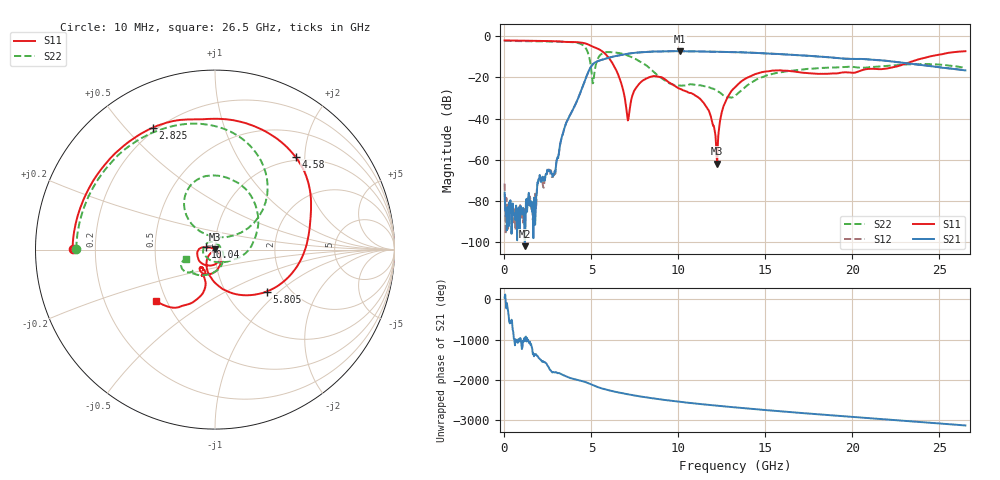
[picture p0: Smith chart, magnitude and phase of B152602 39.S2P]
!  2-Port S-parameters saved by WinCal
! VAR MeasName=S-Parameters (CALIBRATED_DATA) read from VNA (N5242A)
! VAR MeasDate=2016-1-5 16:31:50
! VAR NAME=B152602 39
! VAR FILENAME=B152602 39.S2P
! VAR DATE=2016-1-5 16:31:50
! VAR PHYS_PORTS=1,2
# Hz S DB R 50
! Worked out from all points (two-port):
!   801 points, 10 MHz to 26.5 GHz, reference 50 ohm
!   highest |S21| = -7.22 dB at 10.11 GHz (marker M1); lowest = -102.1 dB at 1.169 GHz (marker M2)
!   |S21| within 3 dB of the highest: 6.073 GHz to 18.7 GHz (12.62 GHz wide, 102 % of centre)
!   lowest |S11| = -61.9 dB at 12.23 GHz (marker M3), VSWR 1.00, Z = 50 + j0.0703 ohm
!   |S11| at or under -10 dB: 5.953 GHz to 24.36 GHz (18.41 GHz wide, 121 % of centre)
!   |S22| runs from -29.8 to -2.2 dB; largest |S21 - S12| = 0.0027
!   S11 on the Smith chart (normalised r, x): 10 MHz: 0.12, +0.00; 2.825 GHz: 0.18, +0.60; 4.58 GHz: 0.93, +1.81; 5.805 GHz: 1.54, -0.83; 10.04 GHz: 0.90, +0.02; 26.5 GHz: 0.44, -0.31
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1e7  -2.02 179.8  -76.03 45.3  -71.65 2.7  -2.24 179.7
1.168938e9  -2.14 156.0  -102.07 48.4  -96.45 -80.0  -2.31 161.9
2.824562e9  -2.35 116.9  -66.88 -3.6  -67.10 -7.7  -2.48 132.6
3.4537e9  -2.70 97.9  -44.51 -93.8  -44.52 -93.7  -2.64 117.6
4.447075e9  -3.09 56.6  -25.63 134.8  -25.64 134.9  -3.94 76.1
4.579525e9  -3.30 49.0  -22.66 118.4  -22.66 118.4  -4.76 65.8
5.109325e9  -5.12 16.7  -13.38 24.7  -13.38 24.9  -22.47 102.4
5.804688e9  -8.61 -39.0  -10.88 -75.1  -10.85 -75.0  -7.80 101.3
6.566275e9  -19.27 -115.3  -9.30 -151.8  -9.30 -151.8  -8.11 70.9
7.096075e9  -40.91 -94.7  -8.47 163.4  -8.46 163.4  -9.37 49.4
7.758325e9  -22.99 -76.0  -7.81 113.4  -7.80 113.4  -12.12 21.2
8.851038e9  -19.63 -158.7  -7.36 43.2  -7.34 43.1  -19.28 -33.3
1.004309e10  -25.42 165.3  -7.23 -21.2  -7.21 -21.2  -23.90 -121.7
1.010931e10  -25.58 165.1  -7.22 -24.6  -7.22 -24.6  -23.94 -126.4
1.150004e10  -32.99 153.1  -7.41 -89.3  -7.41 -89.3  -24.32 157.5
1.222851e10  -61.86 60.5  -7.52 -120.1  -7.52 -120.0  -26.63 113.9
1.259275e10  -34.04 -34.7  -7.58 -135.1  -7.58 -135.2  -28.76 84.0
1.3255e10  -24.78 -56.6  -7.71 -161.6  -7.70 -161.6  -29.01 6.9
1.550665e10  -16.65 -111.6  -8.53 113.6  -8.48 113.5  -18.10 -90.9
1.769208e10  -18.06 -128.9  -9.61 37.7  -9.58 37.8  -15.73 -119.2
2.209604e10  -15.49 -110.6  -12.07 -107.7  -12.01 -107.9  -14.33 -138.4
2.65e10  -7.24 -138.7  -16.57 109.2  -16.56 108.9  -15.28 -161.5
